(* Logix 5000 AddOnInstructionDefinition export Banner_DFG2_DFG3_Param_v4; software revision 33.00; part 2 of 2 *)
(* tags used below, declared in another part *)
   DFG2_DFG3 : Banner_DFG2_DFG3_v4;
   Port_Data : Banner_IOL_Port_v4;
   Port : DINT;
   Local_Control : DINT;
   Command_Being_Processed : BOOL;
   Update_Archive : BOOL;
   Index_Write_Inprocess : DINT;
   Index_Write_Control : DINT;
   Inprocess_Index : DINT;
(* Banner_DFG2_DFG3_Param_v4, continued *)

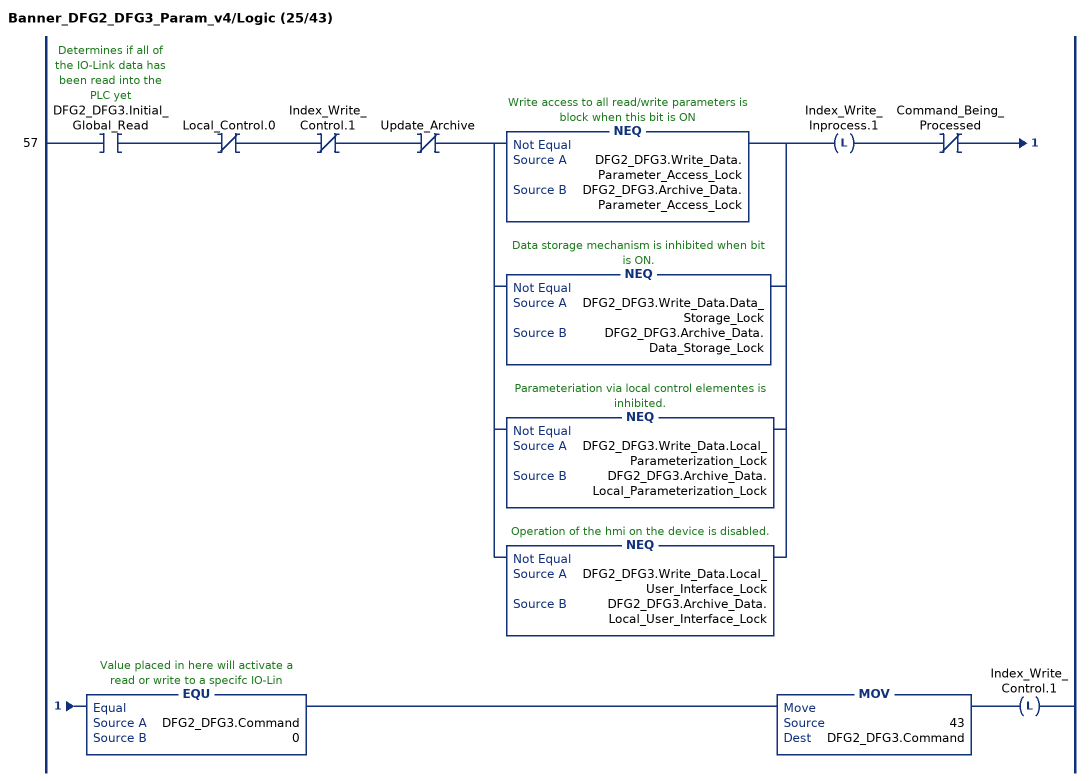
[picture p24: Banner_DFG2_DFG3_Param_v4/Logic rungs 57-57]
   57: XIC(DFG2_DFG3.Initial_Global_Read)XIO(Local_Control.0)XIO(Index_Write_Control.1)XIO(Update_Archive)[NEQ(DFG2_DFG3.Write_Data.Parameter_Access_Lock,DFG2_DFG3.Archive_Data.Parameter_Access_Lock) ,NEQ(DFG2_DFG3.Write_Data.Data_Storage_Lock,DFG2_DFG3.Archive_Data.Data_Storage_Lock) ,NEQ(DFG2_DFG3.Write_Data.Local_Parameterization_Lock,DFG2_DFG3.Archive_Data.Local_Parameterization_Lock) ,NEQ(DFG2_DFG3.Write_Data.Local_User_Interface_Lock,DFG2_DFG3.Archive_Data.Local_User_Interface_Lock) ]OTL(Index_Write_Inprocess.1)XIO(Command_Being_Processed)EQU(DFG2_DFG3.Command,0)MOV(43,DFG2_DFG3.Command)OTL(Index_Write_Control.1);
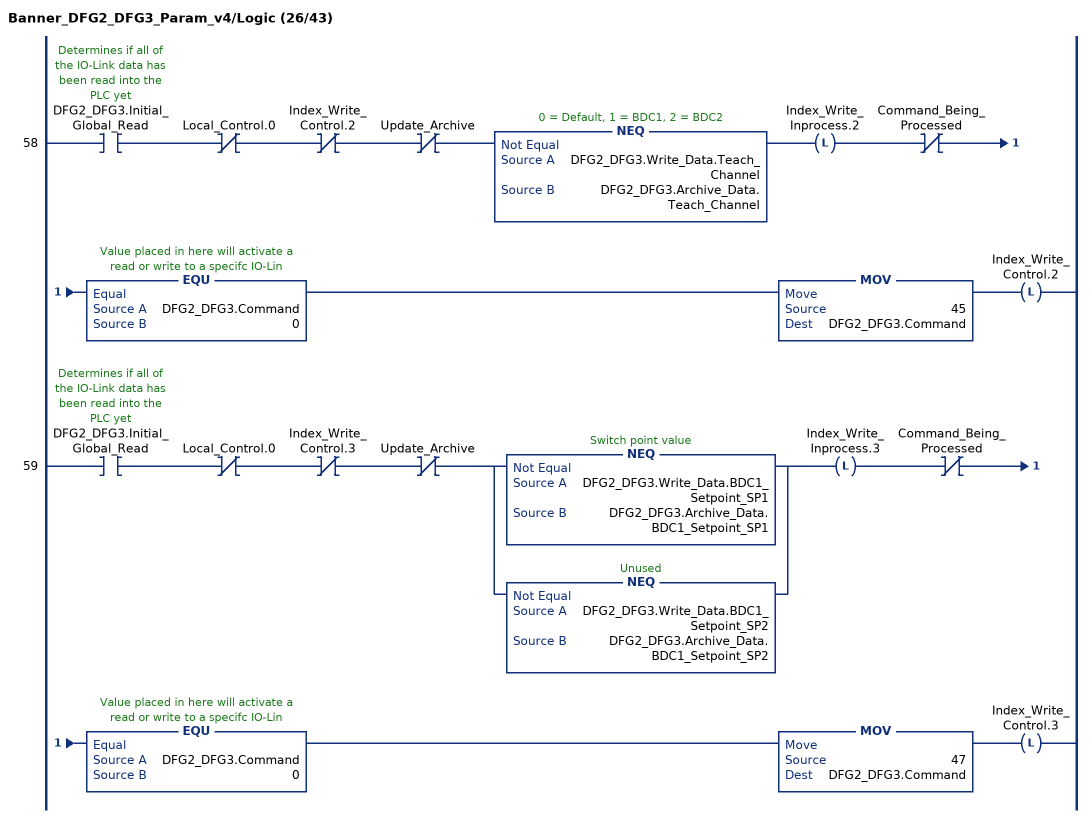
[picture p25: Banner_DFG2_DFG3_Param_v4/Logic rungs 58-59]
   58: XIC(DFG2_DFG3.Initial_Global_Read)XIO(Local_Control.0)XIO(Index_Write_Control.2)XIO(Update_Archive)NEQ(DFG2_DFG3.Write_Data.Teach_Channel,DFG2_DFG3.Archive_Data.Teach_Channel)OTL(Index_Write_Inprocess.2)XIO(Command_Being_Processed)EQU(DFG2_DFG3.Command,0)MOV(45,DFG2_DFG3.Command)OTL(Index_Write_Control.2);
   59: XIC(DFG2_DFG3.Initial_Global_Read)XIO(Local_Control.0)XIO(Index_Write_Control.3)XIO(Update_Archive)[NEQ(DFG2_DFG3.Write_Data.BDC1_Setpoint_SP1,DFG2_DFG3.Archive_Data.BDC1_Setpoint_SP1) ,NEQ(DFG2_DFG3.Write_Data.BDC1_Setpoint_SP2,DFG2_DFG3.Archive_Data.BDC1_Setpoint_SP2) ]OTL(Index_Write_Inprocess.3)XIO(Command_Being_Processed)EQU(DFG2_DFG3.Command,0)MOV(47,DFG2_DFG3.Command)OTL(Index_Write_Control.3);
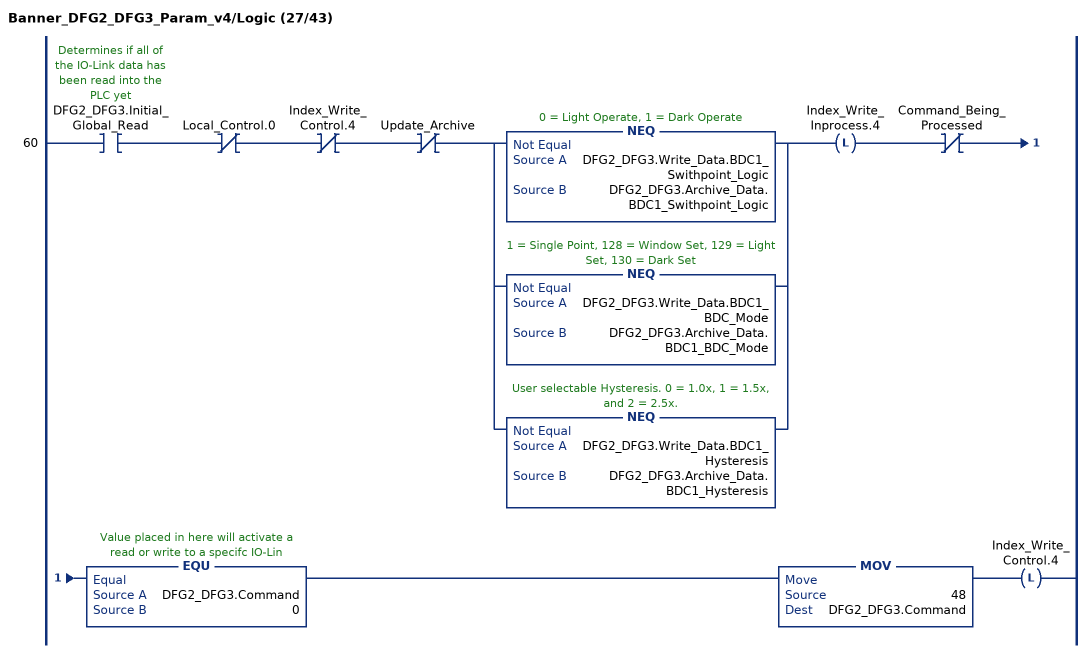
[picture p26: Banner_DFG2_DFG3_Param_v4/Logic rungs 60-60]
   60: XIC(DFG2_DFG3.Initial_Global_Read)XIO(Local_Control.0)XIO(Index_Write_Control.4)XIO(Update_Archive)[NEQ(DFG2_DFG3.Write_Data.BDC1_Swithpoint_Logic,DFG2_DFG3.Archive_Data.BDC1_Swithpoint_Logic) ,NEQ(DFG2_DFG3.Write_Data.BDC1_BDC_Mode,DFG2_DFG3.Archive_Data.BDC1_BDC_Mode) ,NEQ(DFG2_DFG3.Write_Data.BDC1_Hysteresis,DFG2_DFG3.Archive_Data.BDC1_Hysteresis) ]OTL(Index_Write_Inprocess.4)XIO(Command_Being_Processed)EQU(DFG2_DFG3.Command,0)MOV(48,DFG2_DFG3.Command)OTL(Index_Write_Control.4);
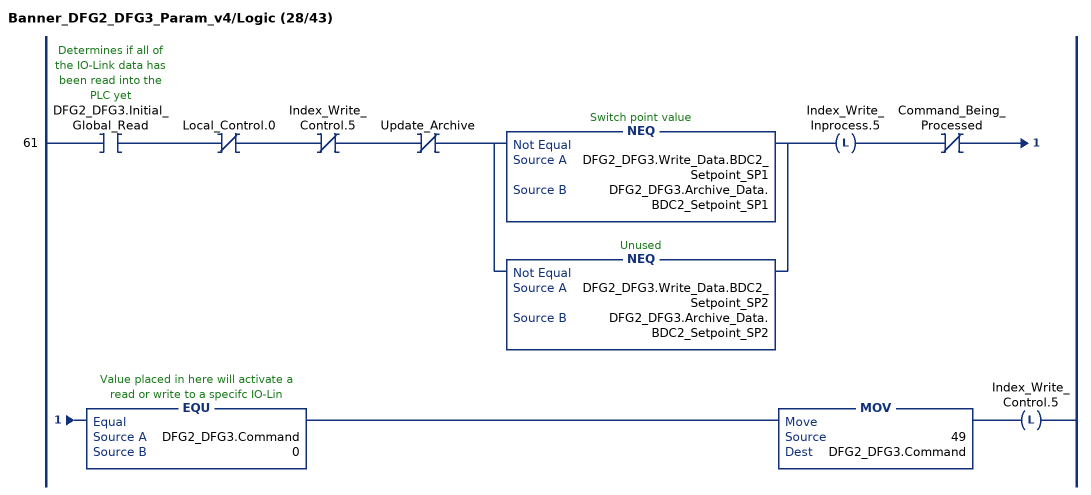
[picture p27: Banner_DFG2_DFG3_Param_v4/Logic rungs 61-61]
   61: XIC(DFG2_DFG3.Initial_Global_Read)XIO(Local_Control.0)XIO(Index_Write_Control.5)XIO(Update_Archive)[NEQ(DFG2_DFG3.Write_Data.BDC2_Setpoint_SP1,DFG2_DFG3.Archive_Data.BDC2_Setpoint_SP1) ,NEQ(DFG2_DFG3.Write_Data.BDC2_Setpoint_SP2,DFG2_DFG3.Archive_Data.BDC2_Setpoint_SP2) ]OTL(Index_Write_Inprocess.5)XIO(Command_Being_Processed)EQU(DFG2_DFG3.Command,0)MOV(49,DFG2_DFG3.Command)OTL(Index_Write_Control.5);
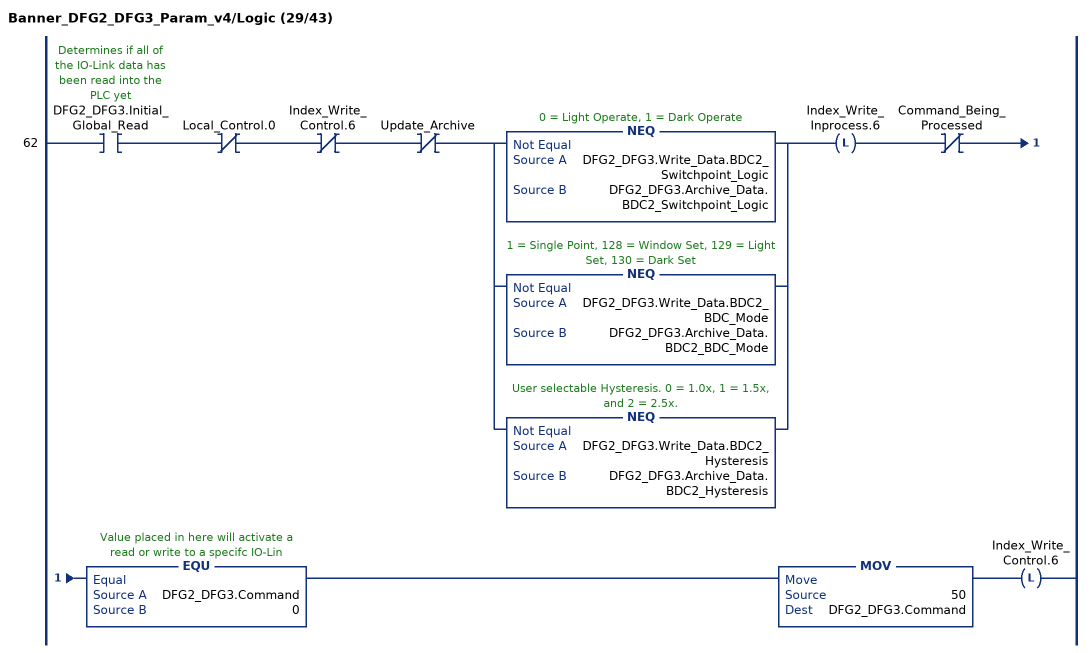
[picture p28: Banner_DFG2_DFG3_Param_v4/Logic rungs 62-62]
   62: XIC(DFG2_DFG3.Initial_Global_Read)XIO(Local_Control.0)XIO(Index_Write_Control.6)XIO(Update_Archive)[NEQ(DFG2_DFG3.Write_Data.BDC2_Switchpoint_Logic,DFG2_DFG3.Archive_Data.BDC2_Switchpoint_Logic) ,NEQ(DFG2_DFG3.Write_Data.BDC2_BDC_Mode,DFG2_DFG3.Archive_Data.BDC2_BDC_Mode) ,NEQ(DFG2_DFG3.Write_Data.BDC2_Hysteresis,DFG2_DFG3.Archive_Data.BDC2_Hysteresis) ]OTL(Index_Write_Inprocess.6)XIO(Command_Being_Processed)EQU(DFG2_DFG3.Command,0)MOV(50,DFG2_DFG3.Command)OTL(Index_Write_Control.6);
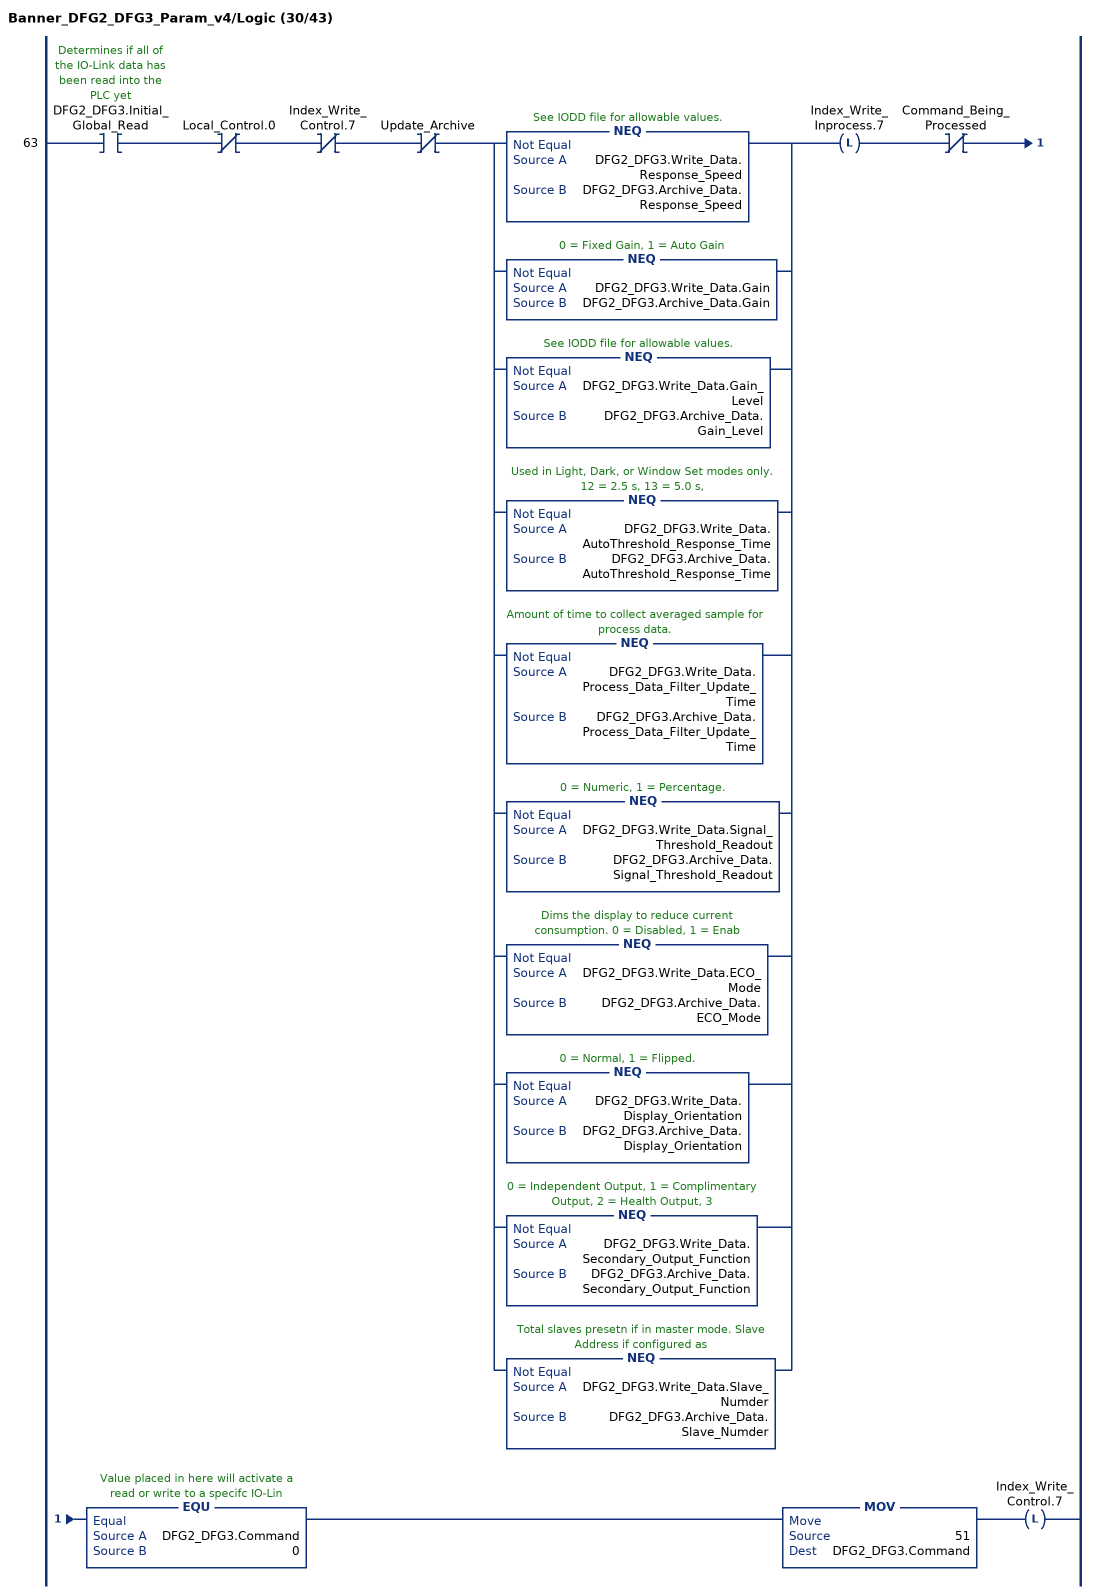
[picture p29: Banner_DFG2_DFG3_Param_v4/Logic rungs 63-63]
   63: XIC(DFG2_DFG3.Initial_Global_Read)XIO(Local_Control.0)XIO(Index_Write_Control.7)XIO(Update_Archive)[NEQ(DFG2_DFG3.Write_Data.Response_Speed,DFG2_DFG3.Archive_Data.Response_Speed) ,NEQ(DFG2_DFG3.Write_Data.Gain,DFG2_DFG3.Archive_Data.Gain) ,NEQ(DFG2_DFG3.Write_Data.Gain_Level,DFG2_DFG3.Archive_Data.Gain_Level) ,NEQ(DFG2_DFG3.Write_Data.AutoThreshold_Response_Time,DFG2_DFG3.Archive_Data.AutoThreshold_Response_Time) ,NEQ(DFG2_DFG3.Write_Data.Process_Data_Filter_Update_Time,DFG2_DFG3.Archive_Data.Process_Data_Filter_Update_Time) ,NEQ(DFG2_DFG3.Write_Data.Signal_Threshold_Readout,DFG2_DFG3.Archive_Data.Signal_Threshold_Readout) ,NEQ(DFG2_DFG3.Write_Data.ECO_Mode,DFG2_DFG3.Archive_Data.ECO_Mode) ,NEQ(DFG2_DFG3.Write_Data.Display_Orientation,DFG2_DFG3.Archive_Data.Display_Orientation) ,NEQ(DFG2_DFG3.Write_Data.Secondary_Output_Function,DFG2_DFG3.Archive_Data.Secondary_Output_Function) ,NEQ(DFG2_DFG3.Write_Data.Slave_Numder,DFG2_DFG3.Archive_Data.Slave_Numder) ]OTL(Index_Write_Inprocess.7)XIO(Command_Being_Processed)EQU(DFG2_DFG3.Command,0)MOV(51,DFG2_DFG3.Command)OTL(Index_Write_Control.7);
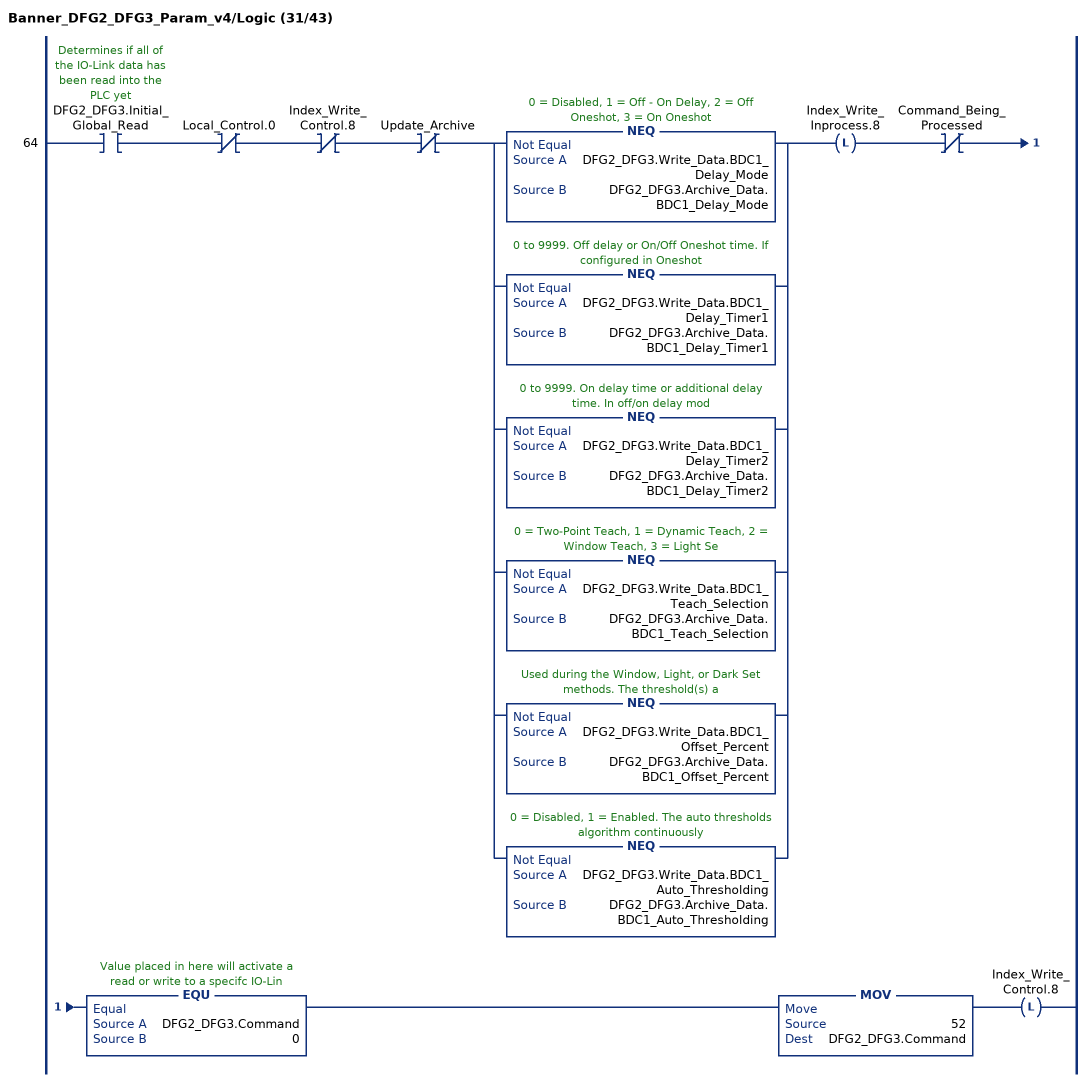
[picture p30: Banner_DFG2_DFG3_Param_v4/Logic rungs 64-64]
   64: XIC(DFG2_DFG3.Initial_Global_Read)XIO(Local_Control.0)XIO(Index_Write_Control.8)XIO(Update_Archive)[NEQ(DFG2_DFG3.Write_Data.BDC1_Delay_Mode,DFG2_DFG3.Archive_Data.BDC1_Delay_Mode) ,NEQ(DFG2_DFG3.Write_Data.BDC1_Delay_Timer1,DFG2_DFG3.Archive_Data.BDC1_Delay_Timer1) ,NEQ(DFG2_DFG3.Write_Data.BDC1_Delay_Timer2,DFG2_DFG3.Archive_Data.BDC1_Delay_Timer2) ,NEQ(DFG2_DFG3.Write_Data.BDC1_Teach_Selection,DFG2_DFG3.Archive_Data.BDC1_Teach_Selection) ,NEQ(DFG2_DFG3.Write_Data.BDC1_Offset_Percent,DFG2_DFG3.Archive_Data.BDC1_Offset_Percent) ,NEQ(DFG2_DFG3.Write_Data.BDC1_Auto_Thresholding,DFG2_DFG3.Archive_Data.BDC1_Auto_Thresholding) ]OTL(Index_Write_Inprocess.8)XIO(Command_Being_Processed)EQU(DFG2_DFG3.Command,0)MOV(52,DFG2_DFG3.Command)OTL(Index_Write_Control.8);
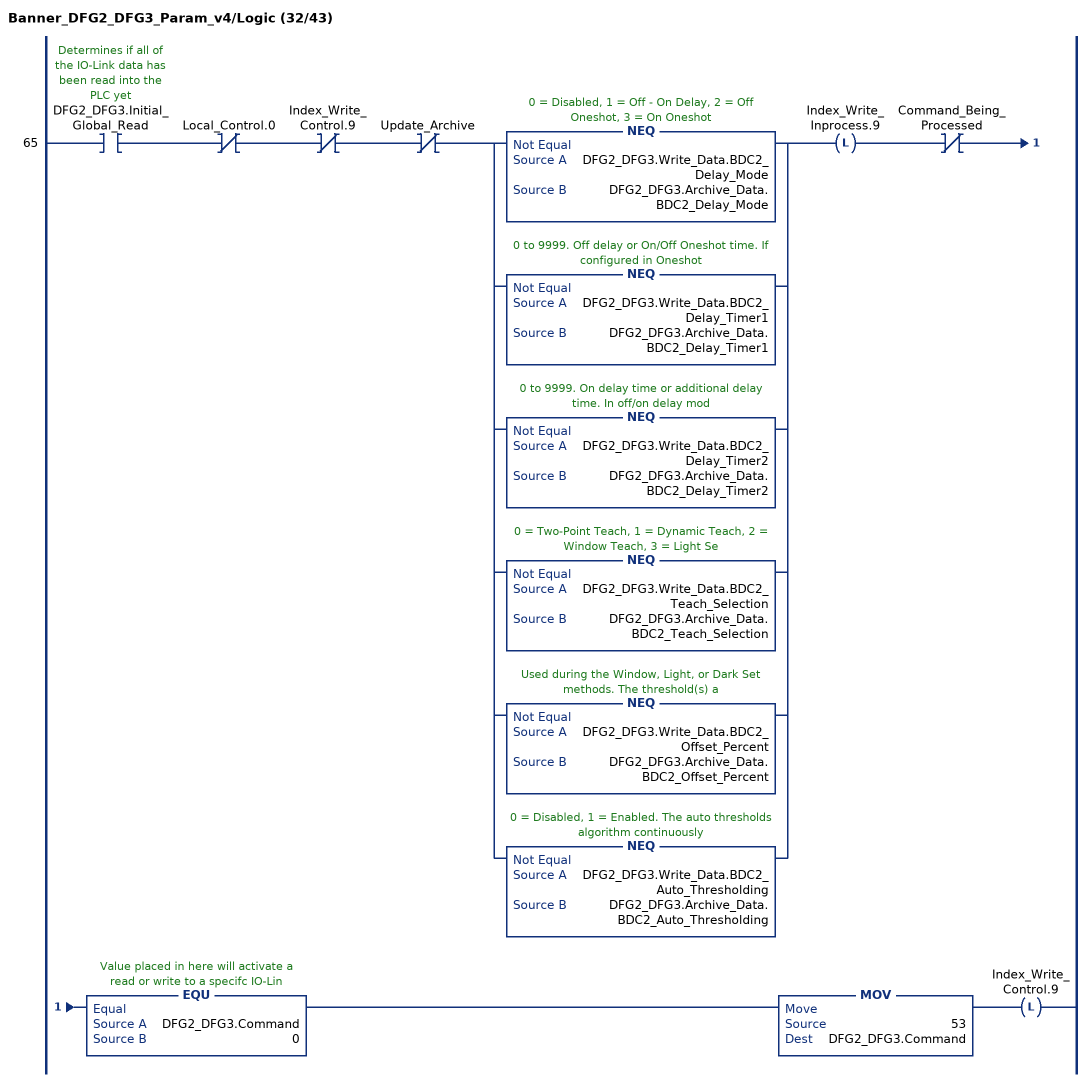
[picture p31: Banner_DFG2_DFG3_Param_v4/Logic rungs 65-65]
   65: XIC(DFG2_DFG3.Initial_Global_Read)XIO(Local_Control.0)XIO(Index_Write_Control.9)XIO(Update_Archive)[NEQ(DFG2_DFG3.Write_Data.BDC2_Delay_Mode,DFG2_DFG3.Archive_Data.BDC2_Delay_Mode) ,NEQ(DFG2_DFG3.Write_Data.BDC2_Delay_Timer1,DFG2_DFG3.Archive_Data.BDC2_Delay_Timer1) ,NEQ(DFG2_DFG3.Write_Data.BDC2_Delay_Timer2,DFG2_DFG3.Archive_Data.BDC2_Delay_Timer2) ,NEQ(DFG2_DFG3.Write_Data.BDC2_Teach_Selection,DFG2_DFG3.Archive_Data.BDC2_Teach_Selection) ,NEQ(DFG2_DFG3.Write_Data.BDC2_Offset_Percent,DFG2_DFG3.Archive_Data.BDC2_Offset_Percent) ,NEQ(DFG2_DFG3.Write_Data.BDC2_Auto_Thresholding,DFG2_DFG3.Archive_Data.BDC2_Auto_Thresholding) ]OTL(Index_Write_Inprocess.9)XIO(Command_Being_Processed)EQU(DFG2_DFG3.Command,0)MOV(53,DFG2_DFG3.Command)OTL(Index_Write_Control.9);
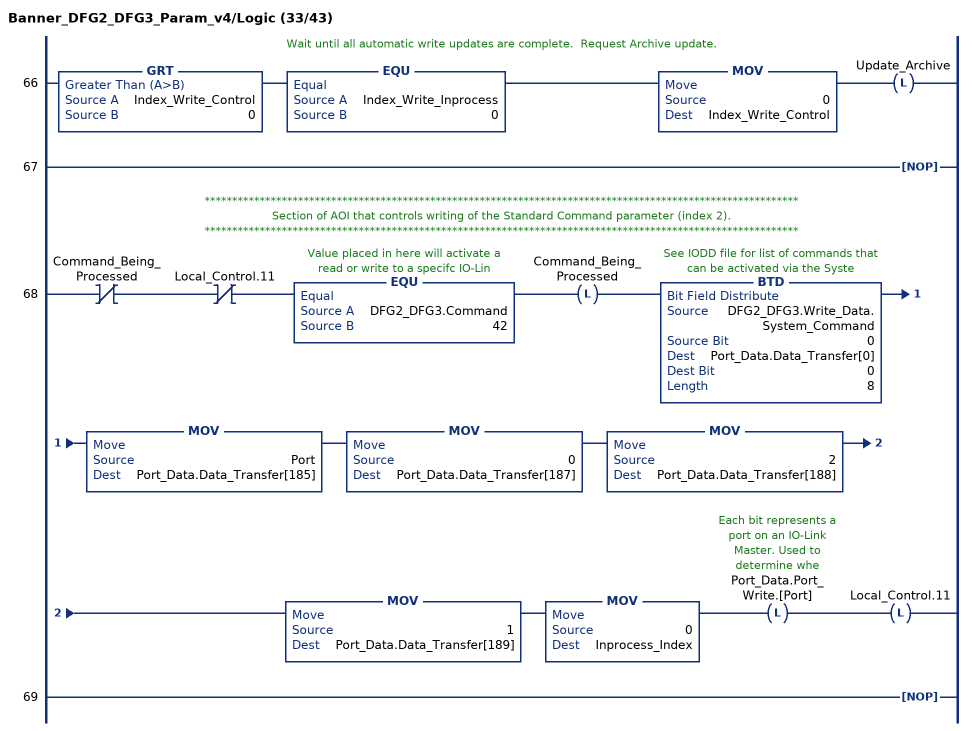
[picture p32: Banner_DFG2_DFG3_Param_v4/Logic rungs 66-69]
   // Wait until all automatic write updates are complete.  Request Archive update.
   66: GRT(Index_Write_Control,0)EQU(Index_Write_Inprocess,0)MOV(0,Index_Write_Control)OTL(Update_Archive);
   67: NOP();
   // ************************************************************************************************************
   // Section of AOI that controls writing of the Standard Command parameter (index 2).
   // ************************************************************************************************************
   68: XIO(Command_Being_Processed)XIO(Local_Control.11)EQU(DFG2_DFG3.Command,42)OTL(Command_Being_Processed)BTD(DFG2_DFG3.Write_Data.System_Command,0,Port_Data.Data_Transfer[0],0,8)MOV(Port,Port_Data.Data_Transfer[185])MOV(0,Port_Data.Data_Transfer[187])MOV(2,Port_Data.Data_Transfer[188])MOV(1,Port_Data.Data_Transfer[189])MOV(0,Inprocess_Index)OTL(Port_Data.Port_Write.[Port])OTL(Local_Control.11);
   69: NOP();
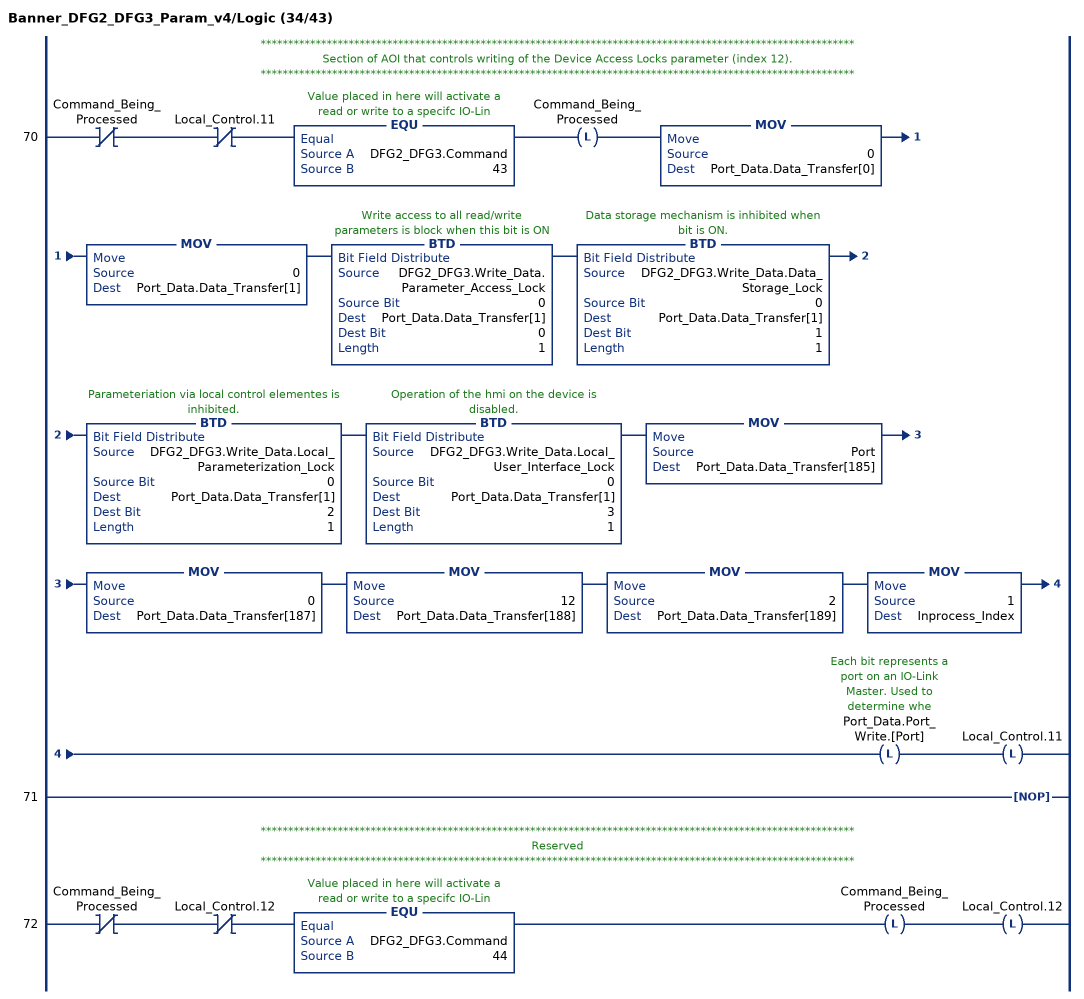
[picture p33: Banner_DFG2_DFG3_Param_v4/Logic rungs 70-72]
   // ************************************************************************************************************
   // Section of AOI that controls writing of the Device Access Locks parameter (index 12).
   // ************************************************************************************************************
   70: XIO(Command_Being_Processed)XIO(Local_Control.11)EQU(DFG2_DFG3.Command,43)OTL(Command_Being_Processed)MOV(0,Port_Data.Data_Transfer[0])MOV(0,Port_Data.Data_Transfer[1])BTD(DFG2_DFG3.Write_Data.Parameter_Access_Lock,0,Port_Data.Data_Transfer[1],0,1)BTD(DFG2_DFG3.Write_Data.Data_Storage_Lock,0,Port_Data.Data_Transfer[1],1,1)BTD(DFG2_DFG3.Write_Data.Local_Parameterization_Lock,0,Port_Data.Data_Transfer[1],2,1)BTD(DFG2_DFG3.Write_Data.Local_User_Interface_Lock,0,Port_Data.Data_Transfer[1],3,1)MOV(Port,Port_Data.Data_Transfer[185])MOV(0,Port_Data.Data_Transfer[187])MOV(12,Port_Data.Data_Transfer[188])MOV(2,Port_Data.Data_Transfer[189])MOV(1,Inprocess_Index)OTL(Port_Data.Port_Write.[Port])OTL(Local_Control.11);
   71: NOP();
   // ************************************************************************************************************
   // Reserved
   // ************************************************************************************************************
   72: XIO(Command_Being_Processed)XIO(Local_Control.12)EQU(DFG2_DFG3.Command,44)OTL(Command_Being_Processed)OTL(Local_Control.12);
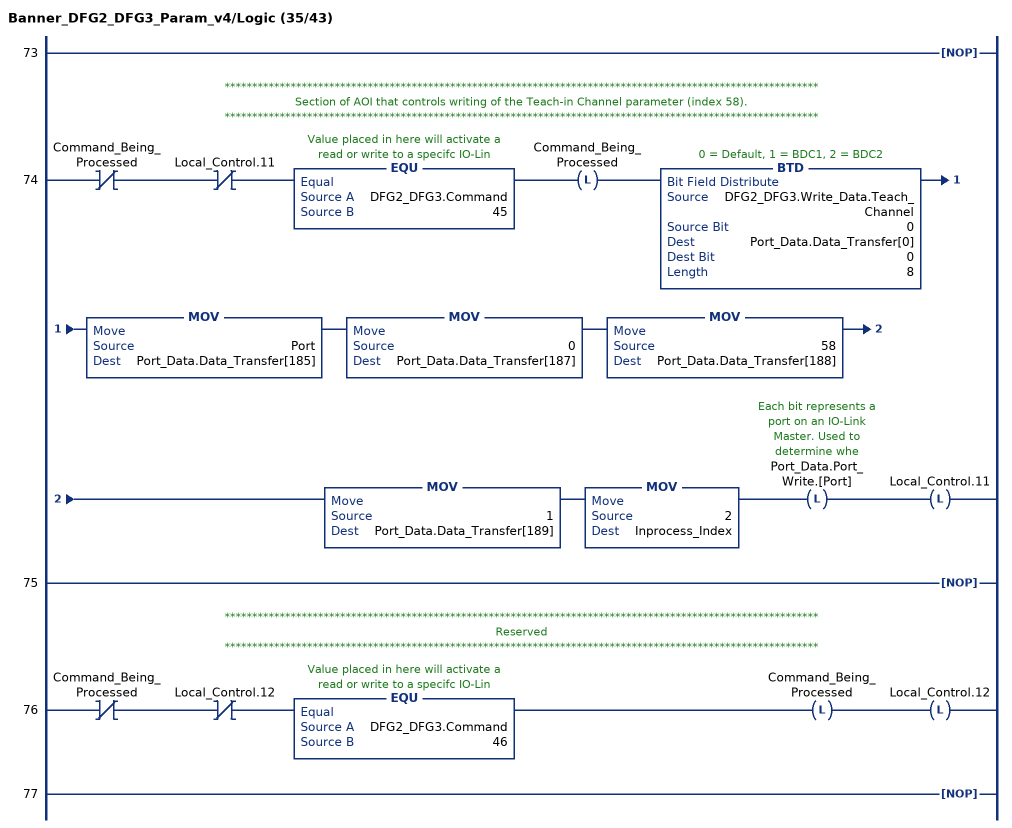
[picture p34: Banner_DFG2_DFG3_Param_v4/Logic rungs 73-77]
   73: NOP();
   // ************************************************************************************************************
   // Section of AOI that controls writing of the Teach-in Channel parameter (index 58).
   // ************************************************************************************************************
   74: XIO(Command_Being_Processed)XIO(Local_Control.11)EQU(DFG2_DFG3.Command,45)OTL(Command_Being_Processed)BTD(DFG2_DFG3.Write_Data.Teach_Channel,0,Port_Data.Data_Transfer[0],0,8)MOV(Port,Port_Data.Data_Transfer[185])MOV(0,Port_Data.Data_Transfer[187])MOV(58,Port_Data.Data_Transfer[188])MOV(1,Port_Data.Data_Transfer[189])MOV(2,Inprocess_Index)OTL(Port_Data.Port_Write.[Port])OTL(Local_Control.11);
   75: NOP();
   // ************************************************************************************************************
   // Reserved
   // ************************************************************************************************************
   76: XIO(Command_Being_Processed)XIO(Local_Control.12)EQU(DFG2_DFG3.Command,46)OTL(Command_Being_Processed)OTL(Local_Control.12);
   77: NOP();
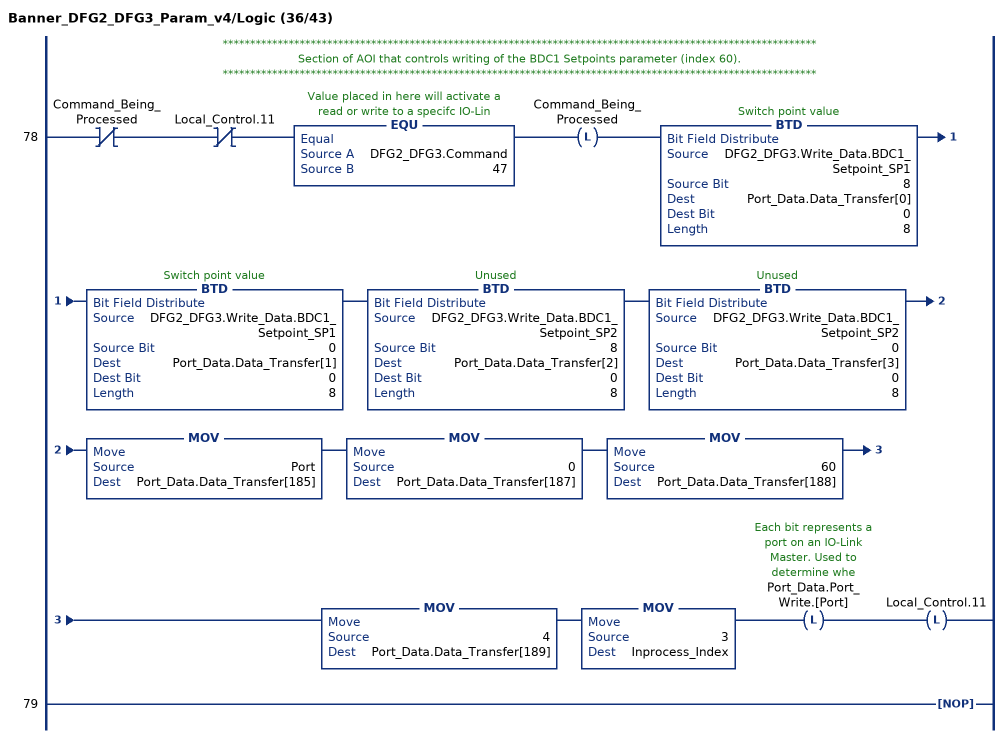
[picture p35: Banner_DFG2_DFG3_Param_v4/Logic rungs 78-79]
   // ************************************************************************************************************
   // Section of AOI that controls writing of the BDC1 Setpoints parameter (index 60).
   // ************************************************************************************************************
   78: XIO(Command_Being_Processed)XIO(Local_Control.11)EQU(DFG2_DFG3.Command,47)OTL(Command_Being_Processed)BTD(DFG2_DFG3.Write_Data.BDC1_Setpoint_SP1,8,Port_Data.Data_Transfer[0],0,8)BTD(DFG2_DFG3.Write_Data.BDC1_Setpoint_SP1,0,Port_Data.Data_Transfer[1],0,8)BTD(DFG2_DFG3.Write_Data.BDC1_Setpoint_SP2,8,Port_Data.Data_Transfer[2],0,8)BTD(DFG2_DFG3.Write_Data.BDC1_Setpoint_SP2,0,Port_Data.Data_Transfer[3],0,8)MOV(Port,Port_Data.Data_Transfer[185])MOV(0,Port_Data.Data_Transfer[187])MOV(60,Port_Data.Data_Transfer[188])MOV(4,Port_Data.Data_Transfer[189])MOV(3,Inprocess_Index)OTL(Port_Data.Port_Write.[Port])OTL(Local_Control.11);
   79: NOP();
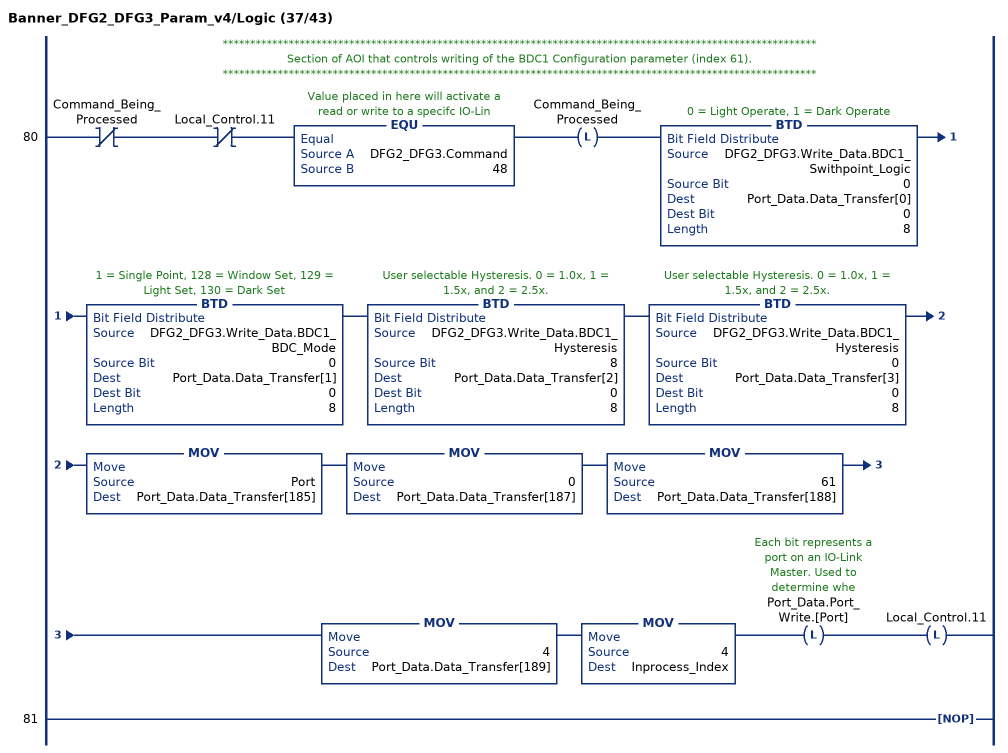
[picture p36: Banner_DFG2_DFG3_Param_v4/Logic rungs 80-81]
   // ************************************************************************************************************
   // Section of AOI that controls writing of the BDC1 Configuration parameter (index 61).
   // ************************************************************************************************************
   80: XIO(Command_Being_Processed)XIO(Local_Control.11)EQU(DFG2_DFG3.Command,48)OTL(Command_Being_Processed)BTD(DFG2_DFG3.Write_Data.BDC1_Swithpoint_Logic,0,Port_Data.Data_Transfer[0],0,8)BTD(DFG2_DFG3.Write_Data.BDC1_BDC_Mode,0,Port_Data.Data_Transfer[1],0,8)BTD(DFG2_DFG3.Write_Data.BDC1_Hysteresis,8,Port_Data.Data_Transfer[2],0,8)BTD(DFG2_DFG3.Write_Data.BDC1_Hysteresis,0,Port_Data.Data_Transfer[3],0,8)MOV(Port,Port_Data.Data_Transfer[185])MOV(0,Port_Data.Data_Transfer[187])MOV(61,Port_Data.Data_Transfer[188])MOV(4,Port_Data.Data_Transfer[189])MOV(4,Inprocess_Index)OTL(Port_Data.Port_Write.[Port])OTL(Local_Control.11);
   81: NOP();
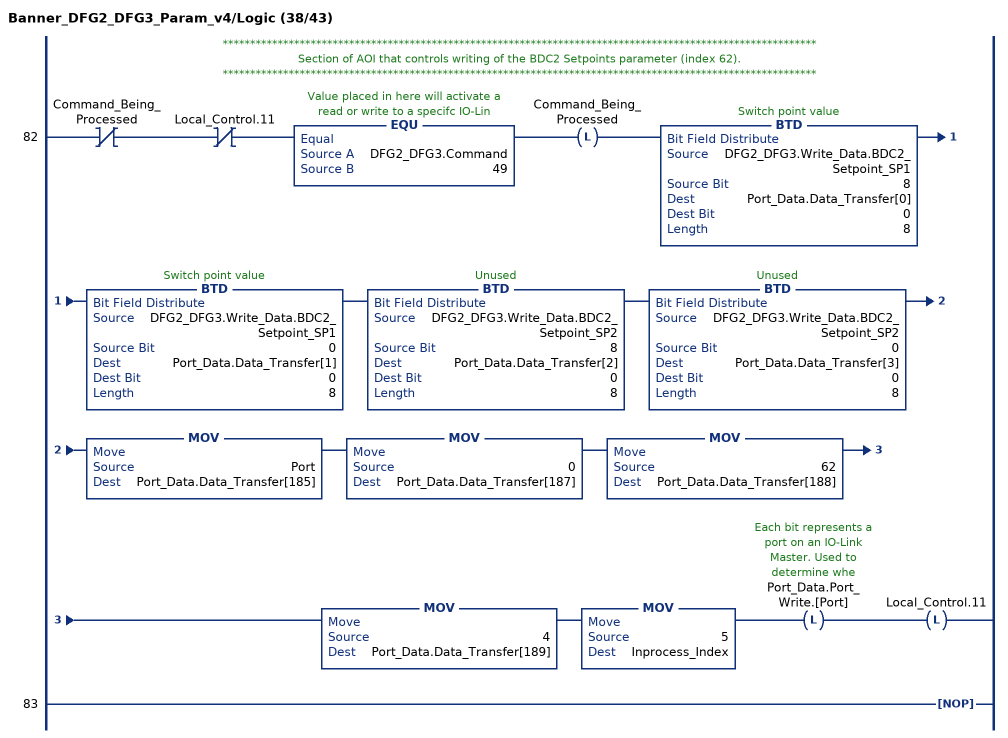
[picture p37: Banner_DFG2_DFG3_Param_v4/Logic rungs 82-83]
   // ************************************************************************************************************
   // Section of AOI that controls writing of the BDC2 Setpoints parameter (index 62).
   // ************************************************************************************************************
   82: XIO(Command_Being_Processed)XIO(Local_Control.11)EQU(DFG2_DFG3.Command,49)OTL(Command_Being_Processed)BTD(DFG2_DFG3.Write_Data.BDC2_Setpoint_SP1,8,Port_Data.Data_Transfer[0],0,8)BTD(DFG2_DFG3.Write_Data.BDC2_Setpoint_SP1,0,Port_Data.Data_Transfer[1],0,8)BTD(DFG2_DFG3.Write_Data.BDC2_Setpoint_SP2,8,Port_Data.Data_Transfer[2],0,8)BTD(DFG2_DFG3.Write_Data.BDC2_Setpoint_SP2,0,Port_Data.Data_Transfer[3],0,8)MOV(Port,Port_Data.Data_Transfer[185])MOV(0,Port_Data.Data_Transfer[187])MOV(62,Port_Data.Data_Transfer[188])MOV(4,Port_Data.Data_Transfer[189])MOV(5,Inprocess_Index)OTL(Port_Data.Port_Write.[Port])OTL(Local_Control.11);
   83: NOP();
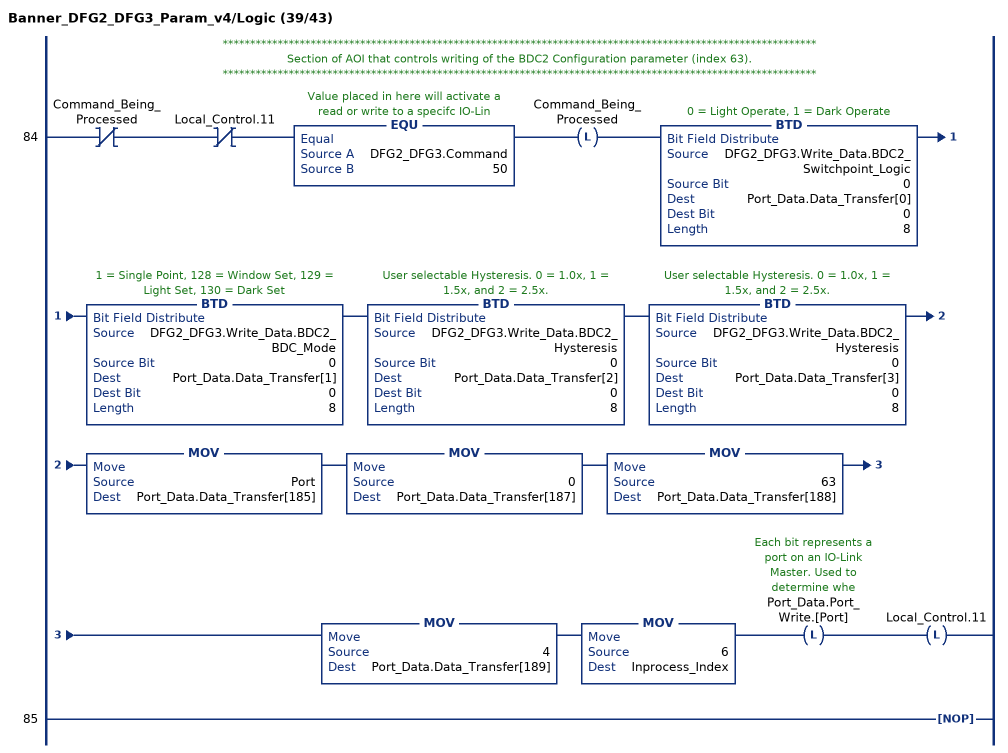
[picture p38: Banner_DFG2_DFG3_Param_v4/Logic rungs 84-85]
   // ************************************************************************************************************
   // Section of AOI that controls writing of the BDC2 Configuration parameter (index 63).
   // ************************************************************************************************************
   84: XIO(Command_Being_Processed)XIO(Local_Control.11)EQU(DFG2_DFG3.Command,50)OTL(Command_Being_Processed)BTD(DFG2_DFG3.Write_Data.BDC2_Switchpoint_Logic,0,Port_Data.Data_Transfer[0],0,8)BTD(DFG2_DFG3.Write_Data.BDC2_BDC_Mode,0,Port_Data.Data_Transfer[1],0,8)BTD(DFG2_DFG3.Write_Data.BDC2_Hysteresis,0,Port_Data.Data_Transfer[2],0,8)BTD(DFG2_DFG3.Write_Data.BDC2_Hysteresis,0,Port_Data.Data_Transfer[3],0,8)MOV(Port,Port_Data.Data_Transfer[185])MOV(0,Port_Data.Data_Transfer[187])MOV(63,Port_Data.Data_Transfer[188])MOV(4,Port_Data.Data_Transfer[189])MOV(6,Inprocess_Index)OTL(Port_Data.Port_Write.[Port])OTL(Local_Control.11);
   85: NOP();
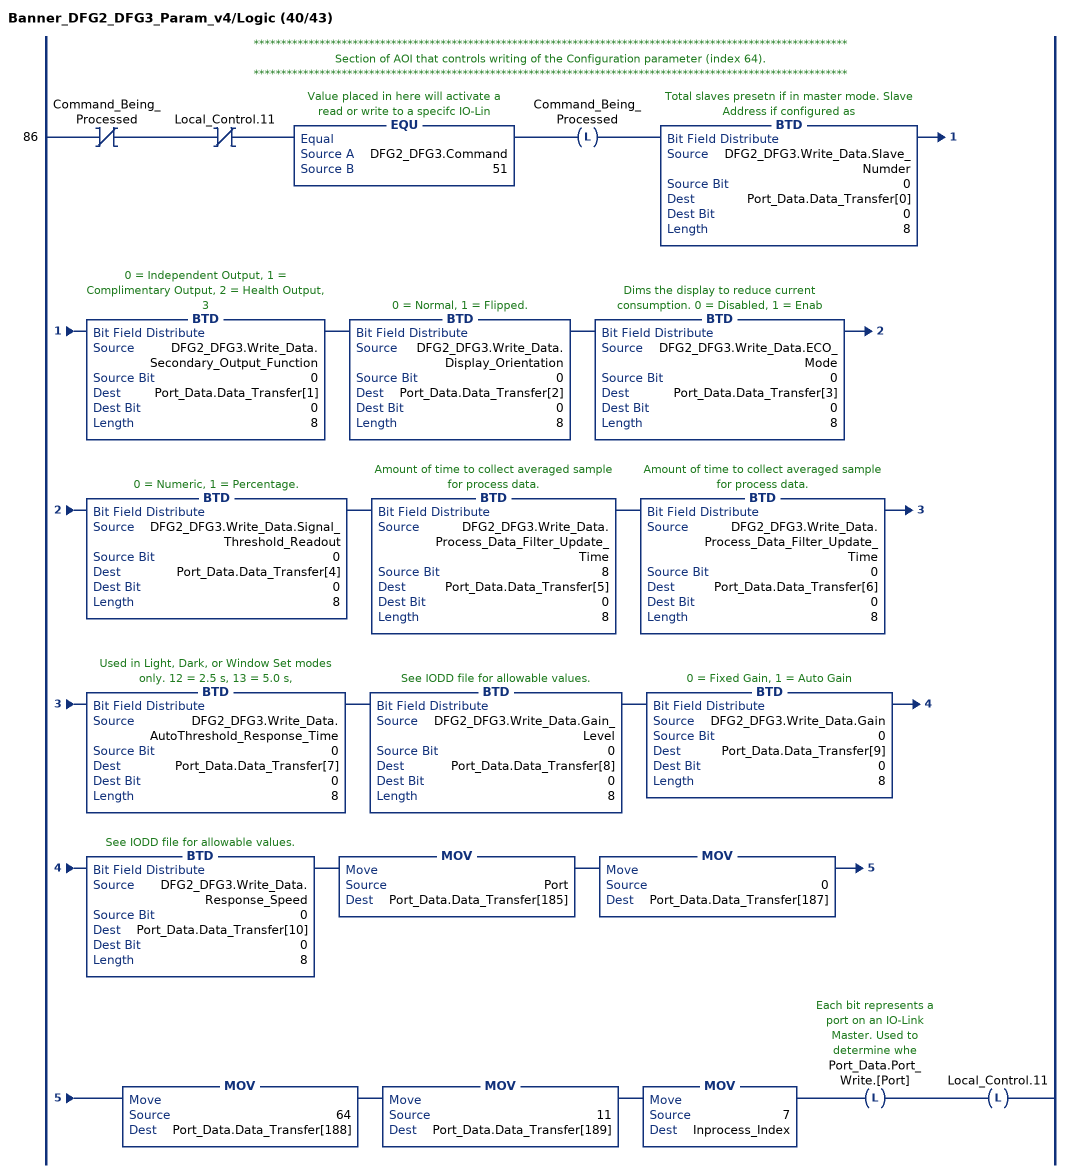
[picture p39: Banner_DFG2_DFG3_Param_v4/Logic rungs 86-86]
   // ************************************************************************************************************
   // Section of AOI that controls writing of the Configuration parameter (index 64).
   // ************************************************************************************************************
   86: XIO(Command_Being_Processed)XIO(Local_Control.11)EQU(DFG2_DFG3.Command,51)OTL(Command_Being_Processed)BTD(DFG2_DFG3.Write_Data.Slave_Numder,0,Port_Data.Data_Transfer[0],0,8)BTD(DFG2_DFG3.Write_Data.Secondary_Output_Function,0,Port_Data.Data_Transfer[1],0,8)BTD(DFG2_DFG3.Write_Data.Display_Orientation,0,Port_Data.Data_Transfer[2],0,8)BTD(DFG2_DFG3.Write_Data.ECO_Mode,0,Port_Data.Data_Transfer[3],0,8)BTD(DFG2_DFG3.Write_Data.Signal_Threshold_Readout,0,Port_Data.Data_Transfer[4],0,8)BTD(DFG2_DFG3.Write_Data.Process_Data_Filter_Update_Time,8,Port_Data.Data_Transfer[5],0,8)BTD(DFG2_DFG3.Write_Data.Process_Data_Filter_Update_Time,0,Port_Data.Data_Transfer[6],0,8)BTD(DFG2_DFG3.Write_Data.AutoThreshold_Response_Time,0,Port_Data.Data_Transfer[7],0,8)BTD(DFG2_DFG3.Write_Data.Gain_Level,0,Port_Data.Data_Transfer[8],0,8)BTD(DFG2_DFG3.Write_Data.Gain,0,Port_Data.Data_Transfer[9],0,8)BTD(DFG2_DFG3.Write_Data.Response_Speed,0,Port_Data.Data_Transfer[10],0,8)MOV(Port,Port_Data.Data_Transfer[185])MOV(0,Port_Data.Data_Transfer[187])MOV(64,Port_Data.Data_Transfer[188])MOV(11,Port_Data.Data_Transfer[189])MOV(7,Inprocess_Index)OTL(Port_Data.Port_Write.[Port])OTL(Local_Control.11);
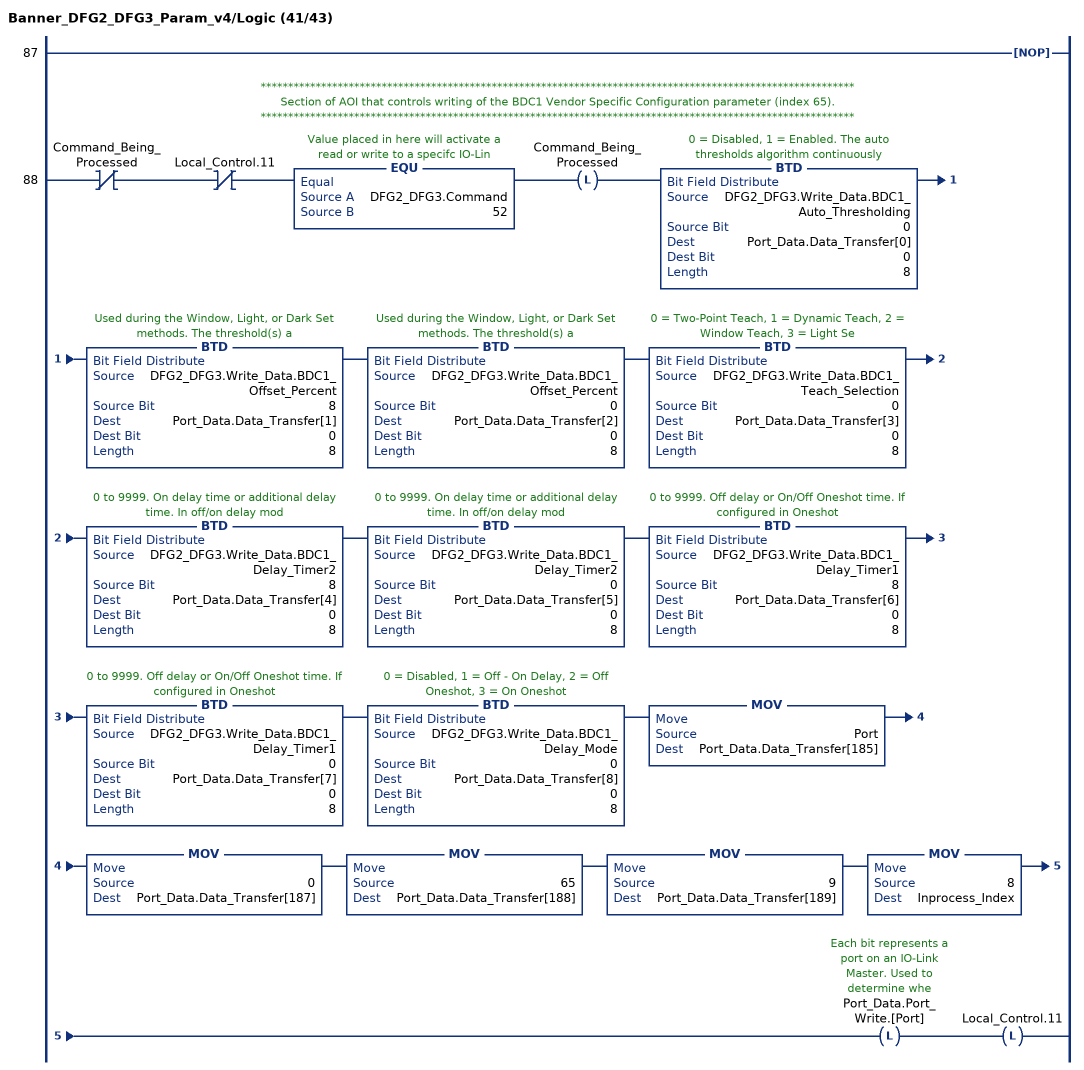
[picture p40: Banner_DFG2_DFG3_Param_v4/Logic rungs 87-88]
   87: NOP();
   // ************************************************************************************************************
   // Section of AOI that controls writing of the BDC1 Vendor Specific Configuration parameter (index 65).
   // ************************************************************************************************************
   88: XIO(Command_Being_Processed)XIO(Local_Control.11)EQU(DFG2_DFG3.Command,52)OTL(Command_Being_Processed)BTD(DFG2_DFG3.Write_Data.BDC1_Auto_Thresholding,0,Port_Data.Data_Transfer[0],0,8)BTD(DFG2_DFG3.Write_Data.BDC1_Offset_Percent,8,Port_Data.Data_Transfer[1],0,8)BTD(DFG2_DFG3.Write_Data.BDC1_Offset_Percent,0,Port_Data.Data_Transfer[2],0,8)BTD(DFG2_DFG3.Write_Data.BDC1_Teach_Selection,0,Port_Data.Data_Transfer[3],0,8)BTD(DFG2_DFG3.Write_Data.BDC1_Delay_Timer2,8,Port_Data.Data_Transfer[4],0,8)BTD(DFG2_DFG3.Write_Data.BDC1_Delay_Timer2,0,Port_Data.Data_Transfer[5],0,8)BTD(DFG2_DFG3.Write_Data.BDC1_Delay_Timer1,8,Port_Data.Data_Transfer[6],0,8)BTD(DFG2_DFG3.Write_Data.BDC1_Delay_Timer1,0,Port_Data.Data_Transfer[7],0,8)BTD(DFG2_DFG3.Write_Data.BDC1_Delay_Mode,0,Port_Data.Data_Transfer[8],0,8)MOV(Port,Port_Data.Data_Transfer[185])MOV(0,Port_Data.Data_Transfer[187])MOV(65,Port_Data.Data_Transfer[188])MOV(9,Port_Data.Data_Transfer[189])MOV(8,Inprocess_Index)OTL(Port_Data.Port_Write.[Port])OTL(Local_Control.11);
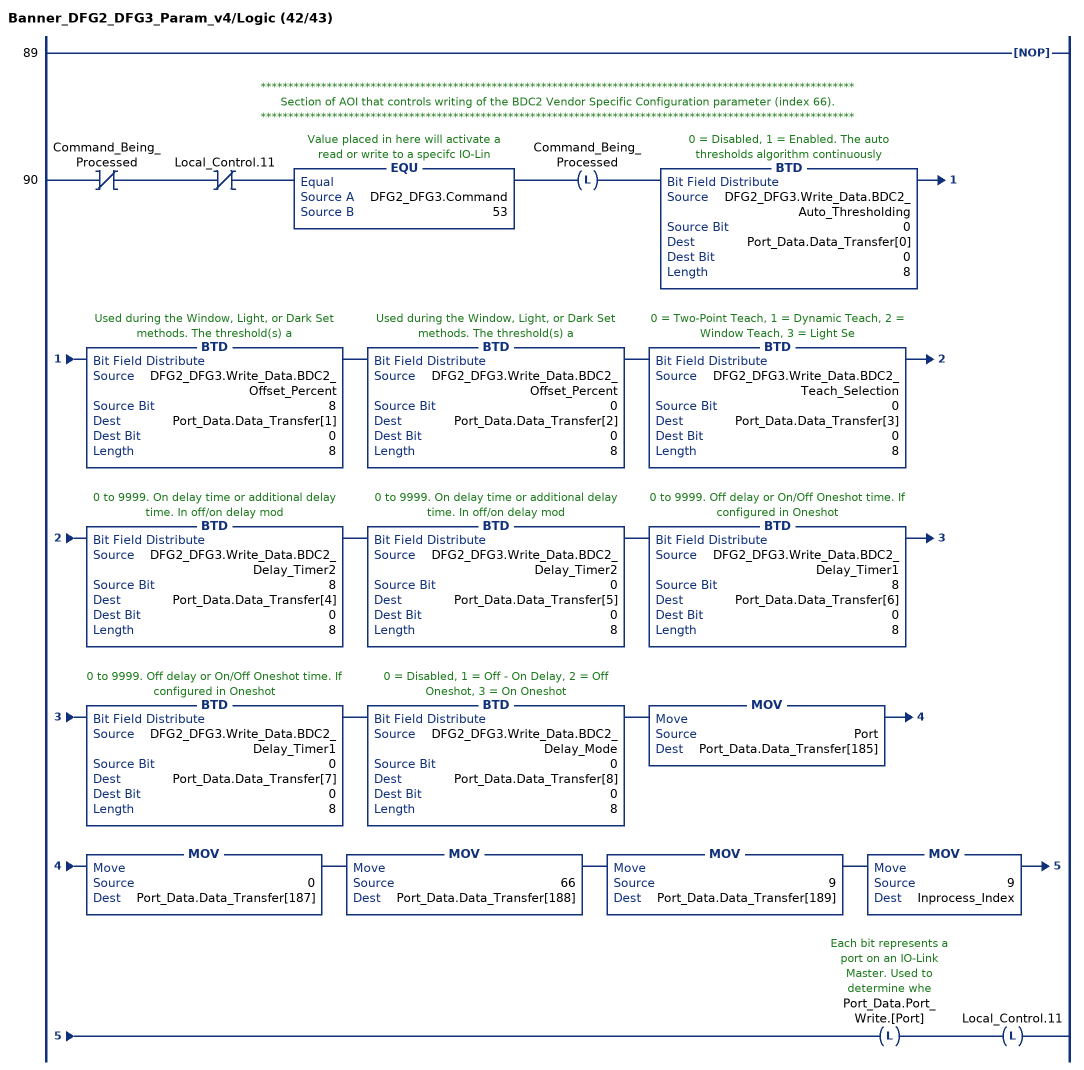
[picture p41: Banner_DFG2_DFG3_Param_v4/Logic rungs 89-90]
   89: NOP();
   // ************************************************************************************************************
   // Section of AOI that controls writing of the BDC2 Vendor Specific Configuration parameter (index 66).
   // ************************************************************************************************************
   90: XIO(Command_Being_Processed)XIO(Local_Control.11)EQU(DFG2_DFG3.Command,53)OTL(Command_Being_Processed)BTD(DFG2_DFG3.Write_Data.BDC2_Auto_Thresholding,0,Port_Data.Data_Transfer[0],0,8)BTD(DFG2_DFG3.Write_Data.BDC2_Offset_Percent,8,Port_Data.Data_Transfer[1],0,8)BTD(DFG2_DFG3.Write_Data.BDC2_Offset_Percent,0,Port_Data.Data_Transfer[2],0,8)BTD(DFG2_DFG3.Write_Data.BDC2_Teach_Selection,0,Port_Data.Data_Transfer[3],0,8)BTD(DFG2_DFG3.Write_Data.BDC2_Delay_Timer2,8,Port_Data.Data_Transfer[4],0,8)BTD(DFG2_DFG3.Write_Data.BDC2_Delay_Timer2,0,Port_Data.Data_Transfer[5],0,8)BTD(DFG2_DFG3.Write_Data.BDC2_Delay_Timer1,8,Port_Data.Data_Transfer[6],0,8)BTD(DFG2_DFG3.Write_Data.BDC2_Delay_Timer1,0,Port_Data.Data_Transfer[7],0,8)BTD(DFG2_DFG3.Write_Data.BDC2_Delay_Mode,0,Port_Data.Data_Transfer[8],0,8)MOV(Port,Port_Data.Data_Transfer[185])MOV(0,Port_Data.Data_Transfer[187])MOV(66,Port_Data.Data_Transfer[188])MOV(9,Port_Data.Data_Transfer[189])MOV(9,Inprocess_Index)OTL(Port_Data.Port_Write.[Port])OTL(Local_Control.11);
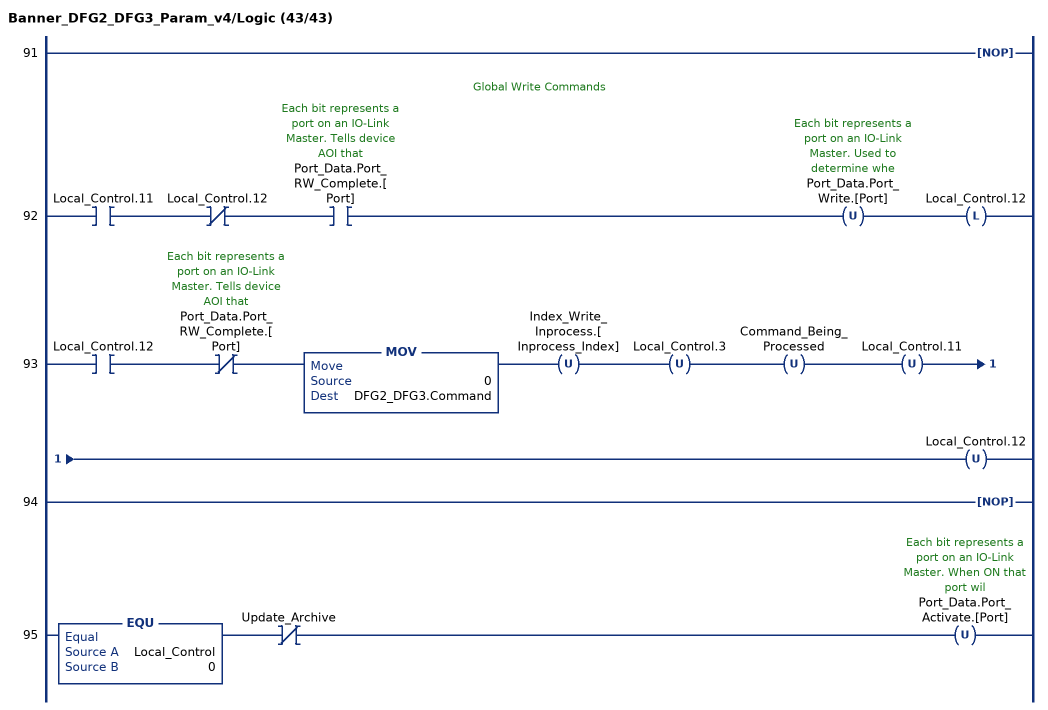
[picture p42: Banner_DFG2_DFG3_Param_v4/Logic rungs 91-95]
   91: NOP();
   // Global Write Commands
   92: XIC(Local_Control.11)XIO(Local_Control.12)XIC(Port_Data.Port_RW_Complete.[Port])OTU(Port_Data.Port_Write.[Port])OTL(Local_Control.12);
   93: XIC(Local_Control.12)XIO(Port_Data.Port_RW_Complete.[Port])MOV(0,DFG2_DFG3.Command)OTU(Index_Write_Inprocess.[Inprocess_Index])OTU(Local_Control.3)OTU(Command_Being_Processed)OTU(Local_Control.11)OTU(Local_Control.12);
   94: NOP();
   95: EQU(Local_Control,0)XIO(Update_Archive)OTU(Port_Data.Port_Activate.[Port]);
END_ROUTINE
END_ADD_ON_INSTRUCTION
